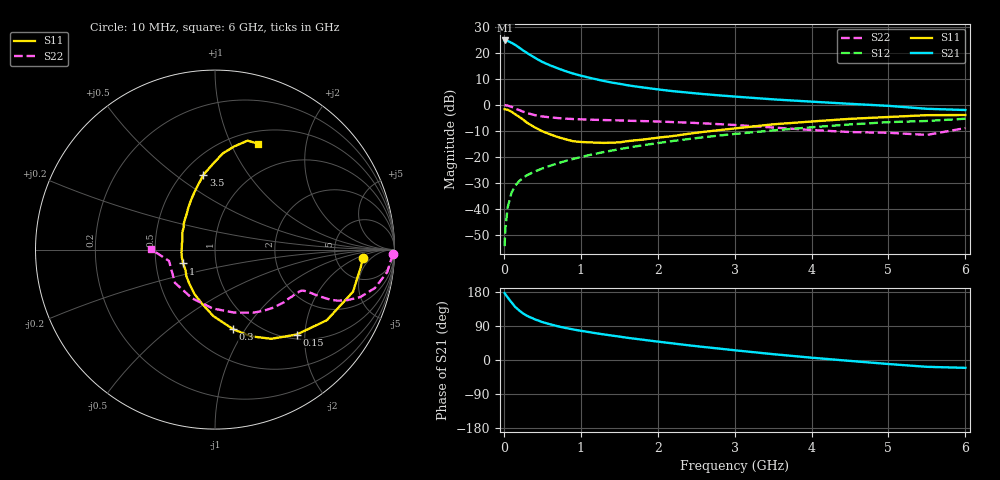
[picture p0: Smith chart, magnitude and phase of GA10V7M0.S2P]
! Infineon Technologies  Discrete & RF Semiconductors
! BF775
! Si NPN RF Bipolar Junction Transistor in SOT23
! VCE = 10 V  IC = 7 mA
! Common Emitter S-Parameters:  May  1996
# GHz  S  MA  R  50
!  f  S11  S21  S12  S22
! GHz  MAG  ANG  MAG  ANG  MAG  ANG  MAG  ANG
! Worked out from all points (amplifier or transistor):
!   36 points, 10 MHz to 6 GHz, reference 50 ohm
!   highest |S21| = 24.8 dB at 20 MHz (marker M1)
!   |S21| within 3 dB of that: start of sweep to 210.7 MHz
!   unconditionally stable (mu >= 1): 760.5 MHz to 2.864 GHz
!   at 250 MHz: K = 0.55, MSG = 24.5 dB, |S12| = -28.1 dB
!   at 1.4 GHz: K = 1.10, MAG = 11.2 dB, |S12| = -17.6 dB
!   at 6 GHz: K = 0.88, MSG = 1.7 dB, |S12| = -5.3 dB
!   S11 on the Smith chart (normalised r, x): 10 MHz: 9.56, -2.84; 150 MHz: 1.09, -1.81; 300 MHz: 0.79, -0.88; 1 GHz: 0.69, -0.11; 3.5 GHz: 0.63, +0.64; 6 GHz: 0.64, +1.28
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0.01  0.8247 -3.3  17.35 176.5  0.0019 95.5  0.991 -1.4
0.02  0.8186 -6.7  17.4 173.3  0.0043 83.3  0.9839 -3.0
0.05  0.8039 -17.0  17.04 165.0  0.0106 81.8  0.9679 -7.4
0.1  0.7369 -32.3  15.7 152.0  0.0204 74.5  0.9166 -13.5
0.15  0.6561 -46.2  14.26 139.5  0.0281 67.5  0.8515 -18.1
0.2  0.5873 -57.8  12.64 130.7  0.034 64.8  0.7916 -20.8
0.25  0.5212 -67.8  11.2 123.0  0.0395 62.4  0.7411 -22.6
0.3  0.4551 -77.1  10.02 116.6  0.0441 61.6  0.6981 -23.5
0.4  0.3707 -91.4  8.134 107.7  0.0519 60.8  0.636 -24.1
0.5  0.3098 -103.6  6.716 100.1  0.0596 61.0  0.598 -24.3
0.6  0.2717 -115.1  5.779 94.3  0.067 61.4  0.5753 -24.4
0.7  0.2403 -126.0  5.061 89.1  0.0748 62.3  0.5572 -24.6
0.8  0.2177 -137.1  4.472 84.6  0.083 62.3  0.5435 -24.9
1  0.1932 -156.5  3.656 77.1  0.0987 63.0  0.5267 -26.2
1.1  0.1898 -166.3  3.361 73.9  0.1071 63.0  0.5208 -27.2
1.3  0.1852 177.9  2.881 67.6  0.1236 62.7  0.5103 -29.1
1.6  0.1993 156.2  2.399 58.8  0.1486 61.8  0.4959 -32.8
2.2  0.2512 129.3  1.836 43.7  0.2018 58.1  0.4663 -42.2
3.5  0.422 98.8  1.277 15.4  0.3222 46.0  0.3665 -73.2
4.5  0.5383 85.3  1.048 -2.4  0.4198 34.1  0.2997 -115.2
5.5  0.6333 73.4  0.84 -18.0  0.4894 18.9  0.2638 -166.2
6  0.6377 67.7  0.796 -20.7  0.5409 14.7  0.3576 179.6
